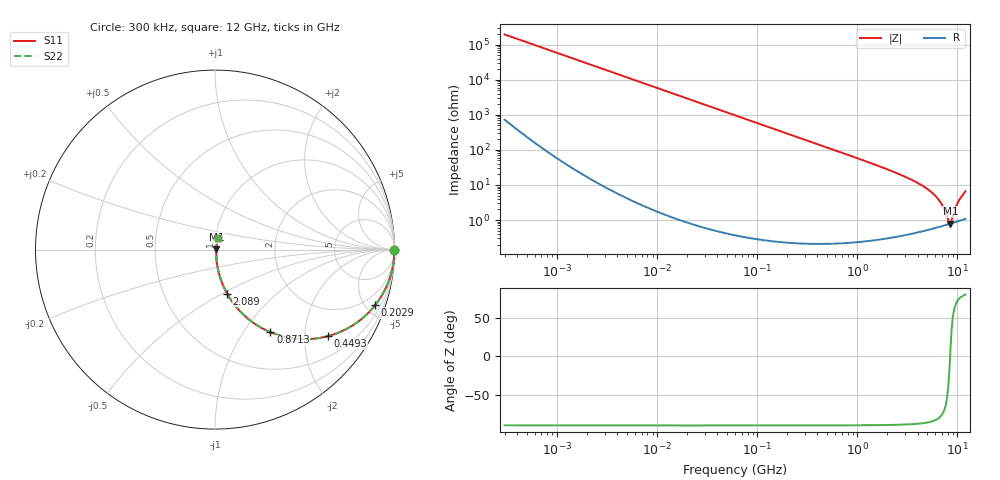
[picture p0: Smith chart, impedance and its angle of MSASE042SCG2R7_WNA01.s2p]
! MSASE042SCG2R7_WNA01  S-PARAMETER MODEL  ( General Type )
! Model Generated by TAIYO YUDEN Corporation (http://www.ty-top.com)
! Version 1.0
! TAIYO YUDEN Control No. 130801
! Copyright(c) 2013 TAIYO YUDEN CO.,LTD. All Rights Reserved.
! Product Description (link to TY-COMPAS)
! https://ds.yuden.co.jp/TYCOMPAS/or/detail?pn=MSASE042SCG2R7AWNA01&u=M
! Products Name : Multilayer Ceramic Capacitors
! Characteristics :
!  Capacitance : 2.7 pF , Rated Voltage : 16V , TCC : CG / C0G
!  Case Size : 0.4 x 0.2 / 0.016 x 0.008 [mm/inch] , Thickness : 0.2 / 0.008 [mm/inch]
!  (Conditions: Temperature = 25 degC , DC Bias Current/Voltage = 0A / 0V)
! External Node Assignments :
!  1  o---| |---o  2
! GND o---------o GND
! Frequency Range : 0.3MHz  -  12000MHz  [ 401 STEP ]
# MHz S RI R 50
! Freq[MHz].  S11 Real  S11 Imag  S21 Real  S21 Imag  S12 Real  S12 Imag  S22 Real  S22 Imag
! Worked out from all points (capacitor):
!   401 points, 300 kHz to 12 GHz, reference 50 ohm
!   read as one part in series: C = 2.71 pF near 316.3 kHz
!   lowest |Z| = 795 mohm at 8.504 GHz (marker M1)
!   series resonance near 8.444 GHz, so ESL is about 130 pH
!   S11 on the Smith chart (normalised r, x): 300 kHz: open; 202.9 MHz: 1.00, -5.79; 449.3 MHz: 1.00, -2.61; 871.3 MHz: 1.00, -1.33; 2.089 GHz: 1.01, -0.53; 12 GHz: 1.02, +0.13
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0.3  1 -0.00051  2.15e-06 0.00051  2.15e-06 0.00051  1 -0.00051
1.769972  1 -0.00301  1.09e-05 0.00301  1.09e-05 0.00301  1 -0.00301
10.44266  0.9997 -0.0178  0.000321 0.0178  0.000321 0.0178  0.9997 -0.0178
60  0.9896 -0.101  0.0104 0.101  0.0104 0.101  0.9896 -0.101
202.9496  0.8932 -0.3085  0.1068 0.3085  0.1068 0.3085  0.8932 -0.3085
353.9943  0.7329 -0.4418  0.2671 0.4418  0.2671 0.4418  0.7329 -0.4418
449.3064  0.6297 -0.4821  0.3703 0.4821  0.3703 0.4821  0.6297 -0.4821
617.4538  0.4728 -0.4981  0.5272 0.4981  0.5272 0.4981  0.4728 -0.4981
871.3074  0.3088 -0.4603  0.6912 0.4603  0.6912 0.4603  0.3088 -0.4603
1331.232  0.1579 -0.3617  0.8421 0.3617  0.8421 0.3617  0.1579 -0.3617
2088.533  0.0678 -0.2456  0.9322 0.2456  0.9322 0.2456  0.0678 -0.2456
3740.715  0.0197 -0.1234  0.9803 0.1234  0.9803 0.1234  0.0197 -0.1234
5420.343  0.00944 -0.063  0.9906 0.063  0.9906 0.063  0.00944 -0.063
6699.894  0.00745 -0.0323  0.9926 0.0323  0.9926 0.0323  0.00745 -0.0323
7254.098  0.00728 -0.0212  0.9927 0.0212  0.9927 0.0212  0.00728 -0.0212
8064.993  0.0075 -0.0066  0.9925 0.0066  0.9925 0.0066  0.0075 -0.0066
8503.825  0.00781 0.0011  0.9922 -0.0011  0.9922 -0.0011  0.00781 0.0011
8732.115  0.00802 0.00538  0.992 -0.00538  0.992 -0.00538  0.00802 0.00538
9708.23  0.00931 0.023  0.9907 -0.023  0.9907 -0.023  0.00931 0.023
10236.47  0.0103 0.0324  0.9897 -0.0324  0.9897 -0.0324  0.0103 0.0324
11380.75  0.0129 0.0517  0.9871 -0.0517  0.9871 -0.0517  0.0129 0.0517
12000  0.0147 0.0631  0.9853 -0.0631  0.9853 -0.0631  0.0147 0.0631
